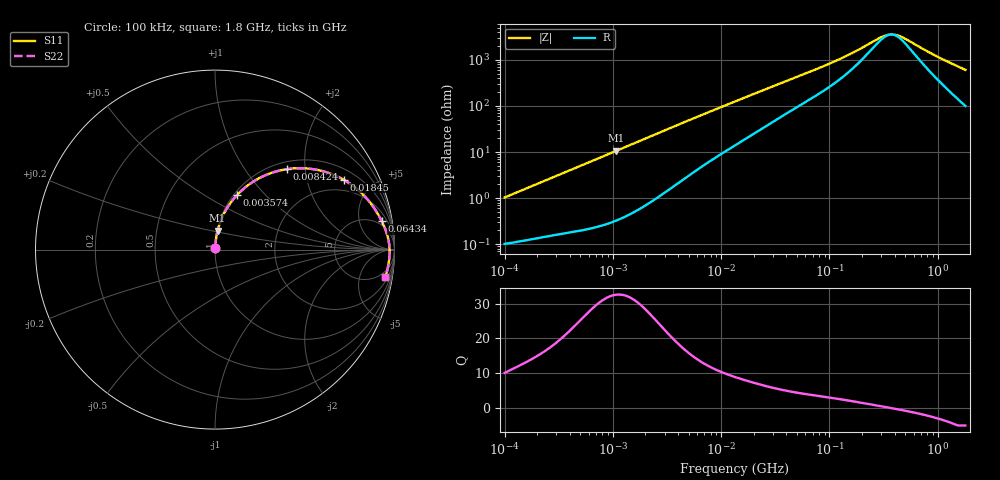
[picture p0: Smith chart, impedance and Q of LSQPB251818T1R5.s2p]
! LSQPB251818T1R5  S-PARAMETER MODEL  ( General Type )
! Model Generated by TAIYO YUDEN Corporation (http://www.ty-top.com)
! Version 2.0
! TAIYO YUDEN Control No. 100810NG19SB-FKC
! Copyright(c) 2009 TAIYO YUDEN CO.,LTD. All Rights Reserved.
! Product Description (link to TY-COMPAS)
! https://ds.yuden.co.jp/TYCOMPAS/or/detail?pn=LSQPB251818T1R5M&u=M
! Products Name : Inductors
! Characteristics :
!  Inductance : 1.5 uH , SRF(min) : 230 MHz , DC Resistance(max) : 0.104 Ohm
!  Rated Current : Saturation :2100 mA , Temp Rise : 1300 mA (40 degC)
!  Case Size : 2.5 x 1.8 / 0.098 x 0.071 [mm/inch] , Thickness : 1.8 / 0.071 [mm/inch]
!  (Conditions: Temperature = 25 degC , DC Bias Current/Voltage = 0A / 0V)
! External Node Assignments :
!  1  o---GGG---o  2
! GND o---------o GND
! Frequency Range : 0.1MHz  -  1800MHz  [ 402 STEP ]
# MHz S RI R 50
! Freq[MHz].  S11 Real  S11 Imag  S21 Real  S21 Imag  S12 Real  S12 Imag  S22 Real  S22 Imag
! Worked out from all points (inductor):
!   401 points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, 100 kHz to 1.8 GHz, reference 50 ohm
!   read as one part in series: L = 1.63 uH near 105 kHz
!   highest Q = 32.6 at 1.076 MHz (marker M1), where L = 1.58 uH
!   self-resonance near 371.3 MHz
!   S11 on the Smith chart (normalised r, x): 100 kHz: 1.00, +0.02; 3.574 MHz: 1.04, +0.70; 8.424 MHz: 1.14, +1.61; 18.45 MHz: 1.44, +3.36; 64.34 MHz: 4, +10; 1.8 GHz: 3, -12
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0.1  0.00113 0.0103  0.9989 -0.0103  0.9989 -0.0103  0.00113 0.0103
0.516129  0.00464 0.0512  0.9954 -0.0512  0.9954 -0.0512  0.00464 0.0512
1.076226  0.0144 0.105  0.9856 -0.105  0.9856 -0.105  0.0144 0.105
1.800136  0.0362 0.1708  0.9638 -0.1708  0.9638 -0.1708  0.0362 0.1708
2.66389  0.0734 0.2409  0.9266 -0.2409  0.9266 -0.2409  0.0734 0.2409
3.574164  0.1218 0.3029  0.8782 -0.3029  0.8782 -0.3029  0.1218 0.3029
5.420303  0.2325 0.3904  0.7675 -0.3904  0.7675 -0.3904  0.2325 0.3904
8.423854  0.4022 0.4485  0.5978 -0.4485  0.5978 -0.4485  0.4022 0.4485
13.41641  0.6004 0.437  0.3996 -0.437  0.3996 -0.437  0.6004 0.437
18.44729  0.7168 0.3894  0.2832 -0.3894  0.2832 -0.3894  0.7168 0.3894
24.15197  0.793 0.3361  0.207 -0.3361  0.207 -0.3361  0.793 0.3361
32.40491  0.8529 0.2758  0.1471 -0.2758  0.1471 -0.2758  0.8529 0.2758
64.33982  0.9286 0.1592  0.0714 -0.1592  0.0714 -0.1592  0.9286 0.1592
69.24595  0.9334 0.1492  0.0666 -0.1492  0.0666 -0.1492  0.9334 0.1492
130.9143  0.9606 0.0781  0.0394 -0.0781  0.0394 -0.0781  0.9606 0.0781
180.0045  0.9671 0.0508  0.0329 -0.0508  0.0329 -0.0508  0.9671 0.0508
293.7968  0.9719 0.0155  0.0281 -0.0155  0.0281 -0.0155  0.9719 0.0155
357.3983  0.9726 0.00251  0.0274 -0.00251  0.0274 -0.00251  0.9726 0.00251
403.9647  0.9728 -0.00557  0.0272 0.00557  0.0272 0.00557  0.9728 -0.00557
467.921  0.9728 -0.0154  0.0272 0.0154  0.0272 0.0154  0.9728 -0.0154
975.7037  0.9679 -0.074  0.0321 0.074  0.0321 0.074  0.9679 -0.074
1800  0.9499 -0.1502  0.0501 0.1502  0.0501 0.1502  0.9499 -0.1502
